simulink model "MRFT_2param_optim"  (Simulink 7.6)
settings: Solver=ode4  SolverMode=SingleTasking  StartTime=0.0  StopTime=20  FixedStep=0.05  RelTol=1e-4  AbsTol=1e-8

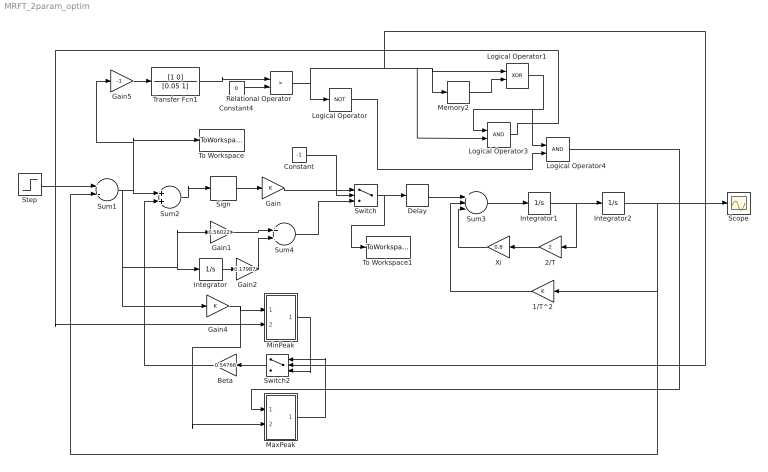
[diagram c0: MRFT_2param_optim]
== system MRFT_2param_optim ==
  1/T^2 : Gain
  2/T : Gain  Gain=2
  Beta : Gain  Gain=0.54766
  Constant : Constant  Value=-1
  Constant4 : Constant  Value=0
  Delay : TransportDelay  DelayTime=2.3
  Gain : Gain
  Gain1 : Gain  Gain=0.56022
  Gain2 : Gain  Gain=0.17987
  Gain4 : Gain
  Gain5 : Gain  Gain=-1
  Integrator : Integrator
  Integrator1 : Integrator
  Integrator2 : Integrator  InitialCondition=0.001
  Logical Operator : Logic  Operator=NOT  Inputs=1
  Logical Operator1 : Logic  Operator=XOR
  Logical Operator3 : Logic
  Logical Operator4 : Logic
  MaxPeak : Subsystem
  Memory2 : Memory
  MinPeak : Subsystem
  Relational Operator : RelationalOperator  Operator=>
  Scope : Scope
  Sign : Signum
  Step : Step  Time=0.1  SampleTime=0.05
  Sum1 : Sum  Inputs=+-
  Sum2 : Sum
  Sum3 : Sum  Inputs=+--
  Sum4 : Sum
  Switch : Switch
  Switch2 : Switch  Threshold=0.5
  To Workspace : ToWorkspace  VariableName=error  SampleTime=-1  SaveFormat=Array
  To Workspace1 : ToWorkspace  VariableName=control  SampleTime=-1  SaveFormat=Array
  Transfer Fcn1 : TransferFcn  Numerator=[1 0]  Denominator=[0.05 1]
  Xi : Gain  Gain=0.8
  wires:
  Memory2/1 -> Logical Operator1/2
  Switch2/1 -> Beta/1
  Logical Operator1/1 -> Logical Operator4/1, Logical Operator3/1
  Logical Operator4/1 -> MaxPeak/1(Cntrl)
  Constant4/1 -> Relational Operator/2
  Relational Operator/1 -> Logical Operator/1, Logical Operator1/1, Memory2/1, Logical Operator3/2, Switch2/2
  Logical Operator3/1 -> MinPeak/2(Cntrl)
  Logical Operator/1 -> Logical Operator4/2
  Sign/1 -> Gain/1
  Gain4/1 -> MinPeak/1(In), MaxPeak/2(In)
  Sum2/1 -> Sign/1
  Sum1/1 -> Sum2/1, Gain5/1, To Workspace/1, Gain4/1, Integrator/1, Gain1/1
  Beta/1 -> Sum2/2
  MaxPeak/1(Out) -> Switch2/1
  MinPeak/1(Out) -> Switch2/3
  Step/1 -> Sum1/1
  Gain5/1 -> Transfer Fcn1/1
  Transfer Fcn1/1 -> Relational Operator/1
  Gain2/1 -> Sum4/2
  Gain1/1 -> Sum4/1
  Integrator/1 -> Gain2/1
  Gain/1 -> Switch/1
  Sum4/1 -> Switch/3
  Constant/1 -> Switch/2
  Sum3/1 -> Integrator1/1
  Integrator1/1 -> Integrator2/1, 2/T/1
  Delay/1 -> Sum3/1
  Integrator2/1 -> Sum1/2, 1/T^2/1, Scope/1
  2/T/1 -> Xi/1
  Xi/1 -> Sum3/3
  1/T^2/1 -> Sum3/2
  Switch/1 -> Delay/1, To Workspace1/1

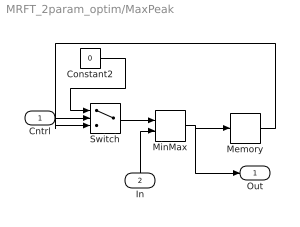
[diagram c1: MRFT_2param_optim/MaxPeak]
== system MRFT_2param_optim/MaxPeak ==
  Cntrl : Inport
  In : Inport  Port=2
  Constant2 : Constant  Value=0
  Memory : Memory
  MinMax : MinMax  Function=max  Inputs=2
  Switch : Switch  Threshold=0.5
  Out : Outport
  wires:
  MinMax/1 -> Memory/1, Out/1
  Switch/1 -> MinMax/1
  Constant2/1 -> Switch/1
  Memory/1 -> Switch/3
  In/1 -> MinMax/2
  Cntrl/1 -> Switch/2

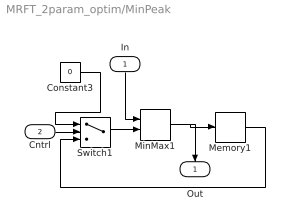
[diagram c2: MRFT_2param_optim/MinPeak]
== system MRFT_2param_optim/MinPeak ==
  In : Inport
  Cntrl : Inport  Port=2
  Constant3 : Constant  Value=0
  Memory1 : Memory
  MinMax1 : MinMax  Inputs=2
  Switch1 : Switch  Threshold=0.5
  Out : Outport
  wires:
  MinMax1/1 -> Memory1/1, Out/1
  Switch1/1 -> MinMax1/2
  Memory1/1 -> Switch1/3
  Constant3/1 -> Switch1/1
  In/1 -> MinMax1/1
  Cntrl/1 -> Switch1/2
